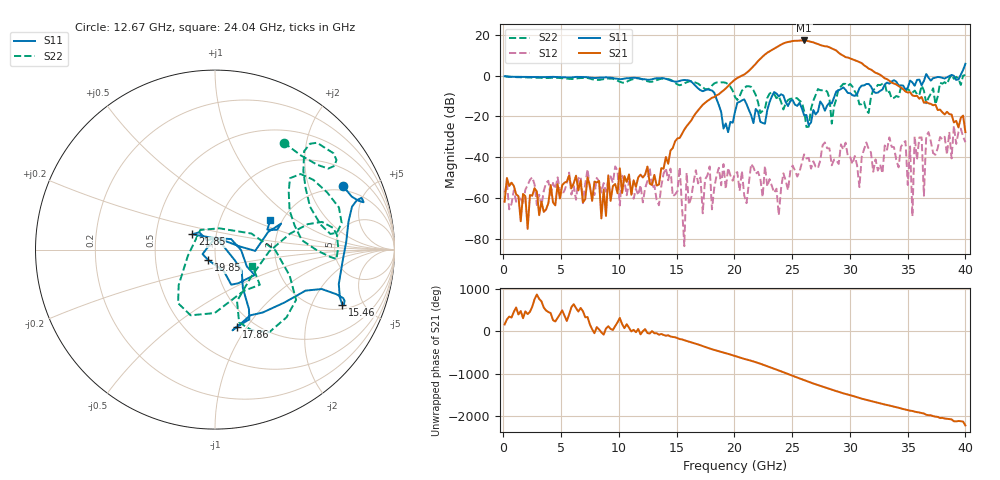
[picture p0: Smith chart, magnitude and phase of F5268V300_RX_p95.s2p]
!S2P File: Measurements: S11,S21,S12,S22
# MHz S  RI  R 50
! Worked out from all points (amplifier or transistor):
!   201 points, 100 MHz to 40 GHz, reference 50 ohm
!   highest |S21| = 17.3 dB at 26.04 GHz (marker M1)
!   |S21| within 3 dB of that: 23.75 GHz to 28.05 GHz (4.303 GHz wide, 16.6 % of centre)
!   unconditionally stable (mu >= 1): start of sweep to 36.45 GHz; 36.76 GHz to 38.6 GHz; 39.14 GHz to 39.42 GHz
!   at 6.684 GHz: K = 1595.55, MAG = -36.0 dB, |S12| = -49.4 dB
!   at 20.05 GHz: K = 138.10, MAG = -1.4 dB, |S12| = -47.9 dB
!   at 40 GHz: K = 119.39, MSG = 2.5 dB, |S12| = -32.6 dB
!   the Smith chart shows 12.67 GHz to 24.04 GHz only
!   S11 on the Smith chart (normalised r, x): 12.67 GHz: 1.76, +3.41; 15.46 GHz: 2.26, -3.44; 17.86 GHz: 0.83, -0.90; 19.85 GHz: 0.92, -0.11; 21.85 GHz: 0.77, +0.13; 24.04 GHz: 1.74, +0.64
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100  -0.9679 0.0461  -0.000771 0.000232  0.00122 0.00055  -0.9808 0.0293
6883  -0.4866 0.7895  -0.000371 0.00068  -0.000635 0.000385  -0.4191 0.7717
12669  0.7129 0.3545  0.00143 -0.00171  -0.00502 -0.0022  0.3826 0.5964
13467  0.8276 0.2641  0.000373 -0.00209  0.000244 -0.000612  0.6657 0.4666
15462  0.7094 -0.3067  -0.0366 0.00689  0.000457 0.000389  0.5883 0.1393
17856  0.1203 -0.4312  0.1805 -0.1877  -0.00121 0.00581  0.4838 0.0525
19851  -0.0369 -0.0591  -0.6385 0.3288  0.00159 0.0021  0.418 0.0889
20050  0.0491 -0.1198  -0.5513 0.5841  0.00396 -0.000776  0.301 -0.0113
21846  -0.1258 0.0856  1.919 -0.3746  -0.00304 0.00246  0.3367 -0.00448
23043  0.2239 -0.00699  -2.387 -3.133  -0.00277 -0.000812  -0.2057 -0.2985
24040  0.3081 0.1628  -3.868 4.294  0.000171 -0.00171  0.208 -0.0891
24639  0.1804 0.00365  2.601 6.186  0.00134 0.000776  -0.00131 0.2525
25237  0.1553 -0.1189  7.148 0.6295  -0.00472 0.000503  -0.1889 0.2121
26035  0.1066 0.00283  1.823 -7.083  -0.01 -0.006  -0.0834 0.109
26833  0.1047 0.0985  -6.036 -2.582  0.00786 0.000933  0.2069 0.1258
27831  0.0753 0.1157  -2.136 4.823  0.0123 0.0193  -0.0345 0.4407
28828  0.3786 0.1646  3.815 1.585  0.00203 0.00817  0.2508 -0.113
29826  0.2821 0.248  1.438 -2.383  0.00697 0.00775  0.2585 0.4998
31023  0.5684 -0.0514  -1.856 -0.8258  0.00506 0.00882  0.037 0.1965
33417  0.5845 -0.2443  0.5608 0.4952  -0.0232 0.02  -0.2221 0.3403
35412  0.4735 -0.4899  0.0111 -0.3263  -0.000101 -0.000338  0.00502 0.3839
40000  1.164 -1.57  0.0136 -0.0387  -0.00514 0.0228  0.2713 -1.003
